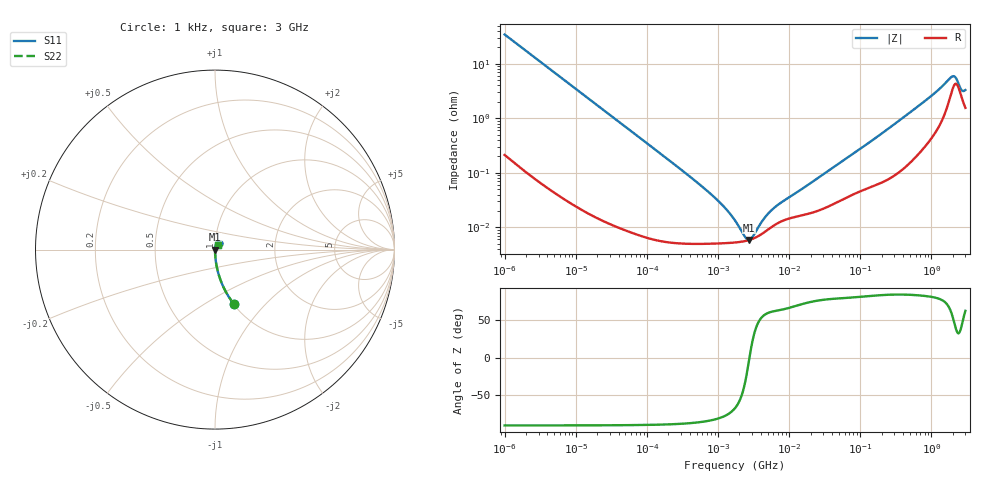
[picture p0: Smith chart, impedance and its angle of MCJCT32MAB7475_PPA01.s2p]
! MCJCT32MAB7475_PPA01  S-PARAMETER MODEL  ( Standard Model )
! Model Generated by TAIYO YUDEN Corporation (http://www.ty-top.com)
! Version 1.0
! TAIYO YUDEN Control No. 220601
! Copyright(c) 2015 TAIYO YUDEN CO.,LTD. All Rights Reserved.
! Product Description (link to TY-COMPAS)
! https://ds.yuden.co.jp/TYCOMPAS/or/detail?pn=MCJCT32MAB7475KPPA01&u=M
! Products Name : Multilayer Ceramic Capacitors
! Characteristics :
!  Capacitance : 4.7 [uF] , Rated Voltage : 25 [V] , TCC : X7R
!  Case Size : 3.2 x 2.5 / 0.126 x 0.098 [mm/inch] , Thickness : 2.5 / 0.098 [mm/inch]
!  (Conditions: Temperature = 25 [degC] , DC Bias Voltage = 0 [V])
! External Node Assignments :
!  1  o---| |---o  2
! GND o---------o GND
! Frequency Range : 1kHz  -  3GHz  [ 401 STEP ]
# MHZ S RI R 50
! Freq[MHz].  S11 Real  S11 Imag  S21 Real  S21 Imag  S12 Real  S12 Imag  S22 Real  S22 Imag
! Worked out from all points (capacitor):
!   401 points, 1 kHz to 3 GHz, reference 50 ohm
!   read as one part in series: C = 4.63 uF near 1.077 kHz
!   lowest |Z| = 5.86 mohm at 2.709 MHz (marker M1)
!   series resonance near 2.766 MHz, so ESL is about 710 pH
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0.001  0.1069 -0.3059  0.8931 0.3059  0.8931 0.3059  0.1069 -0.3059
0.001685  0.0411 -0.1954  0.9589 0.1954  0.9589 0.1954  0.0411 -0.1954
0.00306  0.0132 -0.111  0.9868 0.111  0.9868 0.111  0.0132 -0.111
0.01216  0.00102 -0.0284  0.999 0.0284  0.999 0.0284  0.00102 -0.0284
0.147855  6.22e-05 -0.00236  0.9999 0.00236  0.9999 0.00236  6.22e-05 -0.00236
0.791611  5.03e-05 -0.000406  0.9999 0.000406  0.9999 0.000406  5.03e-05 -0.000406
1.238299  5.13e-05 -0.000226  0.9999 0.000226  0.9999 0.000226  5.13e-05 -0.000226
1.732051  5.28e-05 -0.000123  0.9999 0.000123  0.9999 0.000123  5.28e-05 -0.000123
1.937042  5.36e-05 -9.25e-05  0.9999 9.25e-05  0.9999 9.25e-05  5.36e-05 -9.25e-05
2.087011  5.43e-05 -7.26e-05  0.9999 7.26e-05  0.9999 7.26e-05  5.43e-05 -7.26e-05
2.709407  5.84e-05 -5.21e-06  0.9999 5.21e-06  0.9999 5.21e-06  5.84e-05 -5.21e-06
3.388684  6.54e-05 5.18e-05  0.9999 -5.18e-05  0.9999 -5.18e-05  6.54e-05 5.18e-05
3.651041  6.88e-05 7.09e-05  0.9999 -7.09e-05  0.9999 -7.09e-05  6.88e-05 7.09e-05
4.919932  8.9e-05 0.000146  0.9999 -0.000146  0.9999 -0.000146  8.9e-05 0.000146
6.387174  0.000112 0.00021  0.9999 -0.00021  0.9999 -0.00021  0.000112 0.00021
21.06097  0.000186 0.000653  0.9998 -0.000653  0.9998 -0.000653  0.000186 0.000653
256.0921  0.000824 0.0066  0.9992 -0.0066  0.9992 -0.0066  0.000824 0.0066
944.3747  0.00443 0.0238  0.9956 -0.0238  0.9956 -0.0238  0.00443 0.0238
1917.819  0.0312 0.0461  0.9688 -0.0461  0.9688 -0.0461  0.0312 0.0461
2144.796  0.0421 0.0356  0.9579 -0.0356  0.9579 -0.0356  0.0421 0.0356
2682.519  0.0232 0.0213  0.9768 -0.0213  0.9768 -0.0213  0.0232 0.0213
3000  0.016 0.0281  0.984 -0.0281  0.984 -0.0281  0.016 0.0281
